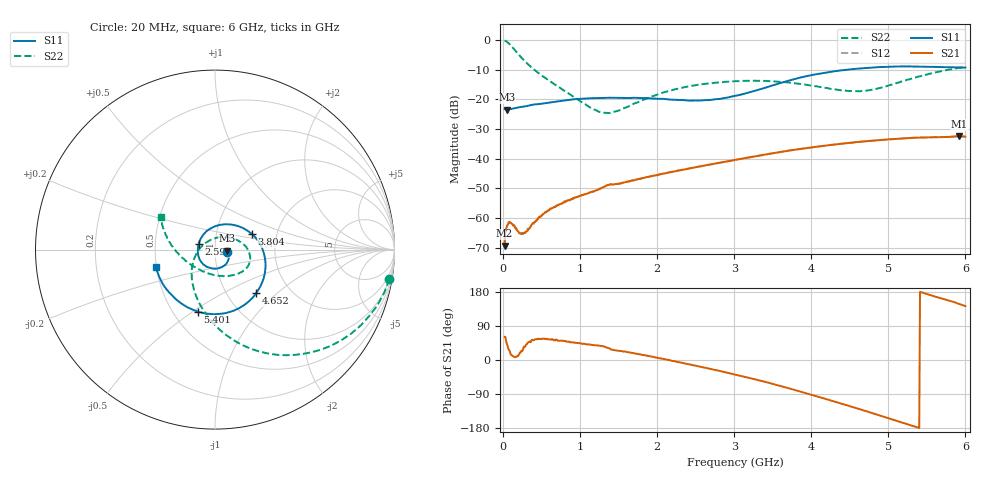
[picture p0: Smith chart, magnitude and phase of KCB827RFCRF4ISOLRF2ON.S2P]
!Agilent Technologies,E5071B,JP1KK00126,A.08.11
!Date: Tue May 06 07:13:16 2014
!Data & Calibration Information:
!Freq	S11:SOLT2(ON)	S21:SOLT2(ON)	S12:SOLT2(ON)	S22:SOLT2(ON)
# Hz S dB R 50
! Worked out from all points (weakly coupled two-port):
!   600 points, 20 MHz to 6 GHz, reference 50 ohm
!   highest |S21| = -32.40 dB at 5.92 GHz (marker M1); lowest = -69.3 dB at 20 MHz (marker M2)
!   lowest |S11| = -23.4 dB at 49.95 MHz (marker M3), VSWR 1.14, Z = 57.2 - j0.646 ohm
!   |S11| at or under -10 dB: start of sweep to 4.459 GHz
!   |S22| runs from -24.6 to -0.1 dB; largest |S21 - S12| = 0.00019
!   S11 on the Smith chart (normalised r, x): 20 MHz: 1.14, -0.03; 2.596 GHz: 0.83, +0.05; 3.804 GHz: 1.49, +0.27; 4.652 GHz: 1.36, -0.74; 5.401 GHz: 0.66, -0.52; 6 GHz: 0.49, -0.11
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2e7  -23.22 -12.7  -69.29 61.1  -69.48 69.4  -0.13 -9.6
4.994992e7  -23.44 -4.8  -62.76 41.6  -62.72 41.8  -0.58 -23.3
7.989983e7  -23.33 -3.4  -61.28 26.4  -61.23 24.4  -1.24 -35.6
1.397997e8  -23.03 -3.5  -62.42 8.6  -62.36 8.4  -2.99 -56.1
2.296494e8  -22.54 -6.1  -65.32 20.4  -65.20 22.1  -5.67 -77.7
3.194992e8  -22.19 -11.3  -64.29 45.2  -63.53 45.0  -8.05 -93.2
5.890484e8  -21.11 -27.1  -57.42 54.7  -57.37 55.3  -13.52 -127.5
1.018331e9  -19.76 -58.2  -52.29 43.4  -52.44 44.0  -20.91 -179.0
1.247947e9  -19.55 -76.7  -50.26 37.9  -50.10 38.2  -24.19 138.3
1.37773e9  -19.44 -87.4  -48.76 31.0  -48.75 30.8  -24.62 109.7
2.016661e9  -19.78 -141.5  -45.39 5.4  -45.35 5.2  -18.24 28.7
2.595693e9  -20.28 161.3  -42.42 -19.3  -42.34 -19.2  -14.83 1.1
3.014992e9  -18.79 110.6  -40.36 -38.5  -40.43 -38.7  -13.87 -14.6
3.444274e9  -15.70 58.8  -38.40 -59.9  -38.41 -60.1  -13.83 -29.9
3.803673e9  -13.00 22.4  -36.89 -80.3  -36.89 -80.4  -14.61 -45.9
4.013322e9  -11.75 4.0  -36.15 -92.5  -36.17 -92.6  -15.41 -58.1
4.332788e9  -10.40 -22.0  -35.12 -111.7  -35.13 -111.6  -16.72 -83.6
4.652254e9  -9.52 -46.7  -34.22 -131.4  -34.23 -131.5  -17.15 -118.9
5.011653e9  -8.97 -73.6  -33.46 -154.0  -33.44 -154.3  -15.22 -158.1
5.401002e9  -8.92 -105.5  -32.88 -179.4  -32.85 -179.6  -12.23 174.4
5.920134e9  -9.24 -155.5  -32.40 147.6  -32.43 147.6  -9.38 152.0
6e9  -9.24 -163.9  -32.54 142.3  -32.55 142.1  -9.05 149.0
